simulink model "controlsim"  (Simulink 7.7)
settings: Solver=ode45  StartTime=0.0  StopTime=inf  RelTol=1e-3
libraries: instrumentlib x2, simulink x1

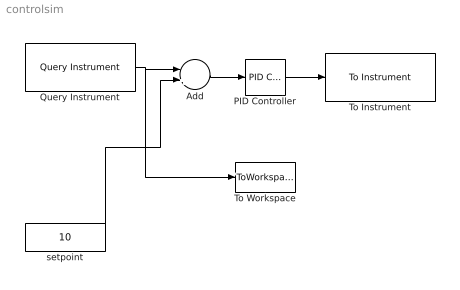
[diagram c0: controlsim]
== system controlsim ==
  Add : Sum  Inputs=-+
  PID Controller : simulink/Continuous/PID Controller  SystemSampleTime=-1  Controller=PID  TimeDomain=Discrete-time  SampleTime=1  IntegratorMethod=Forward Euler  FilterMethod=Forward Euler  Form=Parallel  P=1  I=1  D=1  N=100  InitialConditionSource=internal  InitialConditionForIntegrator=0  InitialConditionForFilter=0  ExternalReset=none  LimitOutput=off  UpperSaturationLimit=inf  LowerSaturationLimit=-inf  LinearizeAsGain=off  AntiWindupMode=none  Kb=1  TrackingMode=off  Kt=1  PParamMin=[]  PParamMax=[]  IParamMin=[]  IParamMax=[]  DParamMin=[]  DParamMax=[]  NParamMin=[]  NParamMax=[]  KbParamMin=[]  KbParamMax=[]  KtParamMin=[]  KtParamMax=[]  POutMin=[]  POutMax=[]  IOutMin=[]  IOutMax=[]  DOutMin=[]  DOutMax=[]  NOutMin=[]  NOutMax=[]  KbOutMin=[]  KbOutMax=[]  KtOutMin=[]  KtOutMax=[]  IntegratorOutMin=[]  IntegratorOutMax=[]  FilterOutMin=[]  FilterOutMax=[]  SumOutMin=[]  SumOutMax=[]  SumI1OutMin=[]  SumI1OutMax=[]  SumI2OutMin=[]  SumI2OutMax=[]  SumI3OutMin=[]  SumI3OutMax=[]  SumDOutMin=[]  SumDOutMax=[]  SaturationOutMin=[]  SaturationOutMax=[]  IntegratorContinuousStateAttributes=''  IntegratorStateMustResolveToSignalObject=off  IntegratorRTWStateStorageClass=Auto  FilterContinuousStateAttributes=''  FilterStateMustResolveToSignalObject=off  FilterRTWStateStorageClass=Auto
  Query Instrument : instrumentlib/Query Instrument  sampleTime=inf  isWorkspaceObject=off  timeout=1  inputBufferSize=50000  protocol=Serial  serialPort=COM2  baudRate=9600  gpibVendor=Advantech  boardIndex=0  primaryAddress=1  secondaryAddress=0  visaVendor=Agilent  visaSerialPort=0  chassisIndex=0  logicalAddress=0  tcpRemoteHost='127.0.0.1'  tcpRemotePort=4500  udpRemoteHost='127.0.0.1'  udpRemotePort=9090  visaTCPBoardIndex=0  visaTCPRemoteHost='127.0.0.1'  usbBoardIndex=0  usbManufID=0  usbModelCode=0  usbSerialNumber=0  initAction=Send ASCII Commands  initCommand='DATA:SOURCE CH1'  initFunction=get  queryCommand='curve?'  responseFormat=ASCII  asciiFormatting='%f,'  precision=8-bit integer  byteOrder=Little endian  valuesToRead=1  removeBytes=off  afterOutputAction=Repeat query for new data  enableFrames=off  frameSize=1
  To Instrument : instrumentlib/To Instrument  sampleTime=inf  isWorkspaceObject=off  timeout=10  inputBufferSize=50000  protocol=Serial  serialPort=COM2  baudRate=9600  gpibVendor=Advantech  boardIndex=0  primaryAddress=1  secondaryAddress=0  visaVendor=Agilent  visaSerialPort=0  chassisIndex=0  logicalAddress=0  tcpRemoteHost='127.0.0.1'  tcpRemotePort=4500  udpRemoteHost='127.0.0.1'  udpRemotePort=9090  visaTCPBoardIndex=0  visaTCPRemoteHost='127.0.0.1'  usbBoardIndex=0  usbManufID=0  usbModelCode=0  usbSerialNumber=0  initAction=Send ASCII Commands  initCommand='DATA:SOURCE CH1'  initFunction=get  command=''  sendFormat=ASCII  asciiFormatting='%f'  precision=8-bit integer  byteOrder=Little endian
  To Workspace : ToWorkspace  VariableName=simout  SampleTime=-1  SaveFormat=Array
  setpoint : Constant  Value=10
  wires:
  setpoint/1 -> Add/2
  Query Instrument/1 -> Add/1, To Workspace/1
  Add/1 -> PID Controller/1
  PID Controller/1 -> To Instrument/1
